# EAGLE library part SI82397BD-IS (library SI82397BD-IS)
Gate Drivers 5 kV 8 V UVLO dual isolated gate drive Source: Datasheet
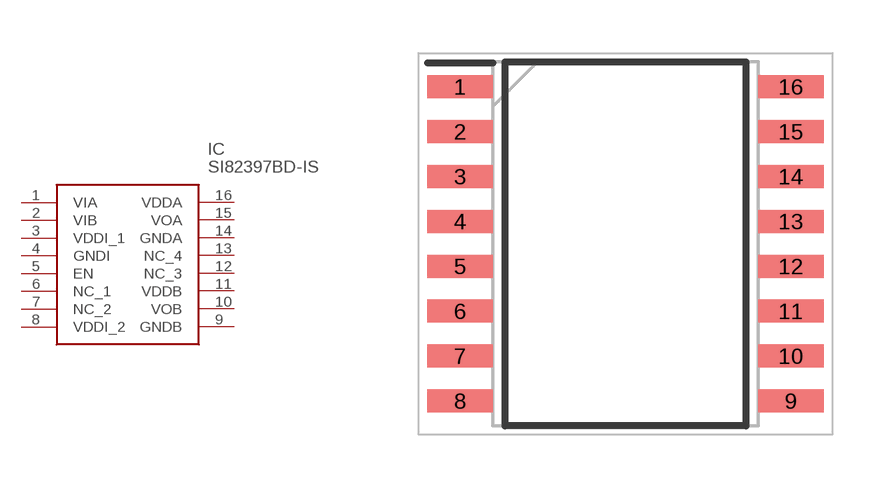
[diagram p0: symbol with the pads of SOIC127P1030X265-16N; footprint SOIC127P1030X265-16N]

Designator prefix IC

## SI82397BD-IS (Description: Gate Drivers 5 kV 8 V UVLO dual isolated gate drive; Height: 2.65mm; Manufacturer_Name: Skyworks; Manufacturer_Part_Number: SI82397BD-IS)  [SOIC127P1030X265-16N]
1  VIA
2  VIB
3  VDDI_1
4  GNDI
5  EN
6  NC_1
7  NC_2
8  VDDI_2
9  GNDB
10  VOB
11  VDDB
12  NC_3
13  NC_4
14  GNDA
15  VOA
16  VDDA

## Footprint SOIC127P1030X265-16N (pad centres in mm)
16-Pin Wide Body SOIC
smd 1.85 x 0.65: 1 -4.675,4.445; 2 -4.675,3.175; 3 -4.675,1.905; 4 -4.675,0.635; 5 -4.675,-0.635; 6 -4.675,-1.905; 7 -4.675,-3.175; 8 -4.675,-4.445; 9 4.675,-4.445; 10 4.675,-3.175; 11 4.675,-1.905; 12 4.675,-0.635; 13 4.675,0.635; 14 4.675,1.905; 15 4.675,3.175; 16 4.675,4.445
